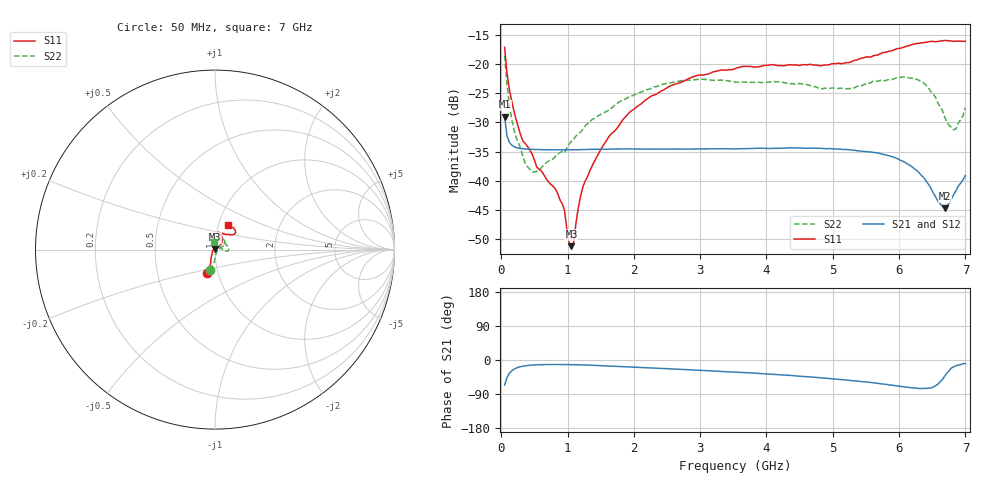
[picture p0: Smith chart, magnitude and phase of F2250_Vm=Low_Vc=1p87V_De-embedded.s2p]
! Integrated Device Technology
! Corporate Headquarters
! 6024 Silver Creek Valley Road
! San Jose, CA 95138  USA
! Phone:  1-408-284-8200
! Toll Free:  1-800-223-1366
! Webpage:  http://www.idt.com/
! Timing and RF Division
! 515 Groton Road, Suite 102
! Westford, MA 01886-6024
! Device:  F2250
! Description: Voltage Variable RF Attenuator
! Frequency:  50.0 -  6000.00 MHz
! Package:  3x3 mm Thin QFN Plastic Package: 16 pin
! Ports:  2 RF, 3 DC
!  Pin  1  = GND
!  Pin  2  = NC
!  Pin  3  = RF1  = Port 1
!  Pin  4  = NC
!  Pin  5  = GND
!  Pin  6  = GND
!  Pin  7  = GND
!  Pin  8  = GND
!  Pin  9  = NC
!  Pin 10  = RF2  = Port 2
!  Pin 11  = NC
!  Pin 12  = GND
!  Pin 13  = GND
!  Pin 14  = VCNTRL
!  Pin 15  = VDD
!  Pin 16  = VMODE
! Vcntrl:  1.870 Volts
! Vmode:  +0.000 Volts
! Vdd:  +3.30  Volts
! Current:  1.185 mA
! Data:  The device was measured on a the F2250 evaluation board which has
!  individual transmission lines to the RF pins.  Data was collected
!  using a calibrated network analyzer.  The evaluation board was
!  de-embedded using a TRL calibration technique.
!  The reference plane is the edge of the package pin.
! Misc:  SN 10
!  Action Tracker AT0258
! Date Measured:  2014-11-26
! Date:  2015-10-15  MJV
! Note:
!  Integrated Device Technology supplies this data as a sample of measured
!  data at the package pin for this product.  Your particular data for this
!  product may vary.
!  Data was taken at 25 degrees C.
!  Integrated Device Technology reserves the right to change this data at anytime.
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# GHz S dB R 50
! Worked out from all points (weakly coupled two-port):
!   201 points, 50 MHz to 7 GHz, reference 50 ohm
!   highest |S21| = -29.04 dB at 50 MHz (marker M1); lowest = -44.7 dB at 6.687 GHz (marker M2)
!   lowest |S11| = -51.2 dB at 1.058 GHz (marker M3), VSWR 1.01, Z = 49.9 + j0.24 ohm
!   |S11| at or under -10 dB: start of sweep to end of sweep
!   |S22| runs from -38.5 to -18.6 dB; largest |S21 - S12| = 5.1e-05
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0.05  -17.17 -108.5  -29.04 -65.9  -29.04 -65.9  -18.56 -103.9
0.1195  -24.20 -111.5  -33.37 -35.8  -33.36 -35.8  -26.80 -88.7
0.189  -28.02 -119.3  -34.14 -24.5  -34.14 -24.5  -31.20 -80.0
0.29325  -32.23 -127.2  -34.47 -17.5  -34.47 -17.4  -34.51 -59.9
0.3975  -34.15 -141.2  -34.59 -14.4  -34.59 -14.4  -37.62 -32.7
0.5365  -37.67 -154.8  -34.66 -12.6  -34.66 -12.6  -38.40 -11.8
0.91875  -43.91 158.1  -34.71 -12.0  -34.71 -12.0  -34.99 9.1
0.9535  -45.02 169.9  -34.71 -12.0  -34.71 -12.0  -35.19 13.2
1.023  -50.74 143.3  -34.70 -12.2  -34.71 -12.2  -33.73 16.0
1.05775  -51.19 119.5  -34.70 -12.3  -34.70 -12.2  -33.25 17.1
1.0925  -50.61 86.3  -34.69 -12.4  -34.70 -12.4  -32.87 16.6
1.162  -44.58 54.5  -34.68 -12.6  -34.68 -12.6  -31.95 14.9
1.2315  -41.03 42.6  -34.65 -13.0  -34.65 -13.0  -31.16 14.2
1.6485  -32.08 41.5  -34.59 -15.8  -34.59 -15.9  -27.70 23.2
2.37825  -24.87 47.1  -34.58 -21.9  -34.58 -22.0  -23.73 32.5
3.525  -20.82 72.4  -34.54 -31.9  -34.55 -31.9  -23.11 59.7
4.7065  -20.18 72.3  -34.40 -45.3  -34.40 -45.3  -23.87 62.9
5.85325  -17.83 40.4  -35.75 -65.6  -35.75 -65.6  -22.67 8.0
6.33975  -16.41 40.9  -39.13 -75.2  -39.13 -75.2  -23.04 -6.0
6.68725  -16.00 48.8  -44.71 -42.6  -44.70 -42.2  -29.07 13.1
6.82625  -16.14 53.5  -42.30 -17.9  -42.25 -17.7  -31.30 51.1
7  -16.13 63.2  -39.10 -9.3  -39.06 -9.3  -27.48 95.3
